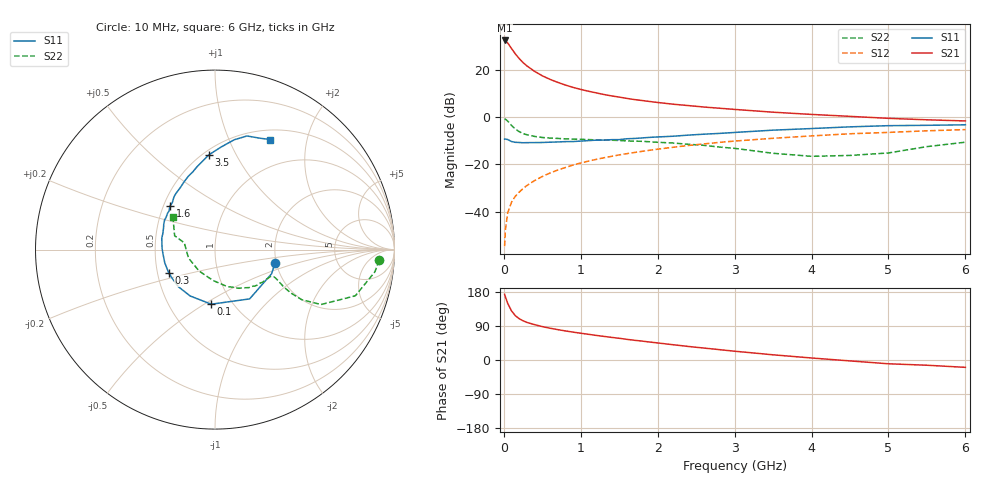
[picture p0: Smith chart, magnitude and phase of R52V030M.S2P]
! SIEMENS Small Signal Semiconductors
! BFR183
! Si NPN RF Bipolar Junction Transistor in SOT23
! VCE = 2 V  IC = 30 mA
! Common Emitter S-Parameters:  May  1996
# GHz  S  MA  R  50
!  f  S11  S21  S12  S22
! GHz  MAG  ANG  MAG  ANG  MAG  ANG  MAG  ANG
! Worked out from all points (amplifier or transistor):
!   36 points, 10 MHz to 6 GHz, reference 50 ohm
!   highest |S21| = 32.3 dB at 10 MHz (marker M1)
!   |S21| within 3 dB of that: start of sweep to 91.62 MHz
!   unconditionally stable (mu >= 1): 358.9 MHz to 2.407 GHz
!   at 250 MHz: K = 0.93, MSG = 26.5 dB, |S12| = -30.1 dB
!   at 1.4 GHz: K = 1.06, MAG = 11.2 dB, |S12| = -16.6 dB
!   at 6 GHz: K = 0.92, MSG = 1.8 dB, |S12| = -5.3 dB
!   S11 on the Smith chart (normalised r, x): 10 MHz: 1.97, -0.33; 100 MHz: 0.80, -0.54; 300 MHz: 0.57, -0.16; 1.6 GHz: 0.54, +0.30; 3.5 GHz: 0.53, +0.78; 6 GHz: 0.62, +1.44
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0.01  0.3421 -12.4  41.07 173.3  0.0019 84.6  0.9167 -3.7
0.02  0.343 -23.0  40.45 166.7  0.0042 75.8  0.8995 -7.9
0.05  0.3357 -54.9  36.43 149.6  0.0095 75.0  0.8235 -18.2
0.1  0.3049 -93.9  27.78 129.6  0.0161 70.1  0.6653 -27.4
0.15  0.2931 -118.2  21.38 116.9  0.0215 69.3  0.5586 -30.0
0.2  0.2906 -134.5  17.07 109.0  0.0262 70.5  0.4918 -29.8
0.25  0.2873 -145.7  14.03 103.4  0.0311 70.6  0.4485 -28.9
0.3  0.2886 -153.3  11.96 99.2  0.0361 72.0  0.4227 -27.9
0.4  0.2894 -165.3  9.168 93.3  0.0458 73.0  0.3902 -26.1
0.5  0.2908 -175.4  7.385 88.1  0.0558 73.8  0.3705 -25.1
0.6  0.2948 178.8  6.223 83.9  0.0661 73.7  0.3608 -24.8
0.7  0.2985 172.5  5.38 80.2  0.0764 73.4  0.3542 -25.2
0.8  0.3032 167.7  4.721 76.7  0.0864 72.2  0.347 -25.7
0.9  0.3043 162.6  4.212 73.6  0.0973 71.8  0.3421 -26.3
1.1  0.3186 153.7  3.494 67.8  0.1178 70.4  0.3348 -28.9
1.3  0.327 146.2  2.985 62.3  0.1385 68.4  0.3268 -31.4
1.6  0.3485 136.1  2.467 54.5  0.1692 65.2  0.314 -36.4
2.2  0.3938 119.8  1.863 40.3  0.2307 58.3  0.2835 -48.4
3.5  0.529 93.7  1.264 13.7  0.3564 40.8  0.1722 -93.8
4.5  0.6211 80.1  1.033 -2.4  0.4441 27.4  0.1551 -162.3
5.5  0.6688 68.2  0.874 -13.8  0.5124 15.2  0.2379 161.0
6  0.686 63.3  0.827 -19.4  0.5437 7.5  0.2949 142.6
